|   TEXAS INSTRUMENTS INCORPORATED
|   Standard Linear and Logic
|   IBIS Model of SN74LVTH162373
|   3.3-V ABT 16-BIT TRANSPARENT D-TYPE LATCHES
|   WITH 3-STATE OUTPUTS
|   TSSOP 48-pin package (DGG)
|   SSOP 48-pin package (DL)
[IBIS Ver]   3.2
[Comment char]   |_char
[File Name]   sn74lvth162373.ibs
[File Rev]   1.1 | a_die
[Date]   10/08/03
[Source]   File originated at Texas Instruments, Inc
[Notes]   The following is an IBIS list for SN74LVTH162373.
|   - All test data contained in this file are derived from
|   actual measurement.
|   - Non-monotonic data in ground-clamp due to bus-hold
|   - Power clamp data deleted in input models.
|   - Non-monotonic data in pullup data due to resistor at output.
|   - End point warning due to AC and DC mismatch.
|   - File created by Nobuhisa Ohtsubo, TIJ SLL Product Engineering.
|*   Property of Texas Instruments Incorporated.  Unauthorized   *
|*   reproduction and/or distribution is strictly prohibited.   *
|*   This product is protected under copyright law.   *
|*   Created 1998, (C) Copyright 1998, Texas Instruments Inc.,   *
|*   All Rights Reserved   *
|*   UNLESS THERE IS A SIGNED, WRITTEN AGREEMENT TO THE   *
|*   CONTRARY, TEXAS INSTRUMENTS ("TI") IS PROVIDING THE SPICE   *
|*   MODELS "AS IS" AND WITHOUT ANY WARRANTY, EXPRESSED OR   *
|*   IMPLIED.  TI assumes no liability for:   *
|*   1) the accuracy of the IBIS models provided to your   *
|*   company;   *
|*   2) the proper functioning of these IBIS models in your   *
|*   design or for any resulting applications; or   *
|*   3) infringement of patents, copyrights or intellectual   *
|*   property rights resulting from your use of these   *
|*   IBIS models.   *
|*   TI provides IBIS Models as a service to our customers.   *
|*   You and your company shall not distribute, sell or give   *
|*   these models to anyone else without prior written   *
|*   permission from TI.   *
|*   TI reserves the right to make changes to our products or   *
|*   to discontinue any semiconductor product or service   *
|*   without notice, and advises our customers to obtain the   *
|*   latest version of relevant information to verify, before   *
|*   placing orders, that the information being relied on is   *
|*   current.   *
|*   Please be aware that your receipt and use of the IBIS   *
|*   information provided shall serve as acceptance of these   *
|*   terms and conditions.  If you do not accept these terms,   *
|*   you should return or destroy the IBIS models and any   *
|*   other accompanying information immediately.   *
|   TSSOP PACKAGE (DGG)
[Component]   LVTH162373_DGG
[manufacturer]   Texas Instruments, Inc.
[Package]
|   typ   min   max
R_pkg   0.044   0.038   0.051
L_pkg   3.019nH   2.486nH   4.099nH
C_pkg   0.507pF   0.334pF   0.809pF
[Pin] signal_name   model_name   R_pin   L_pin   C_pin
1   1NOE   LVTH162373_CTRL  0.041   4.017nH   0.759pF
2   1Q1   LVTH162373_OUT   0.042   3.737nH   0.792pF
3   1Q2   LVTH162373_OUT   0.042   3.48nH   0.661pF
4   GND   GND   0.038   3.131nH   0.575pF
5   1Q3   LVTH162373_OUT   0.047   3.122nH   0.566pF
6   1Q4   LVTH162373_OUT   0.043   2.948nH   0.504pF
7   VCC   POWER   0.045   2.845nH   0.397pF
8   1Q5   LVTH162373_OUT   0.049   2.835nH   0.394pF
9   1Q6   LVTH162373_OUT   0.048   2.715nH   0.378pF
10   GND   GND   0.050   2.664nH   0.363pF
11   1Q7   LVTH162373_OUT   0.050   2.585nH   0.348pF
12   1Q8   LVTH162373_OUT   0.049   2.55nH   0.337pF
13   2Q1   LVTH162373_OUT   0.049   2.541nH   0.336pF
14   2Q2   LVTH162373_OUT   0.050   2.574nH   0.348pF
15   GND   GND   0.049   2.618nH   0.359pF
16   2Q3   LVTH162373_OUT   0.046   2.671nH   0.375pF
17   2Q4   LVTH162373_OUT   0.045   2.754nH   0.389pF
18   VCC   POWER   0.044   2.823nH   0.450pF
19   2Q5   LVTH162373_OUT   0.042   2.968nH   0.503pF
20   2Q6   LVTH162373_OUT   0.051   3.108nH   0.535pF
21   GND   GND   0.042   3.175nH   0.587pF
22   2Q7   LVTH162373_OUT   0.041   3.449nH   0.678pF
23   2Q8   LVTH162373_OUT   0.044   3.766nH   0.804pF
24   2NOE   LVTH162373_CTRL  0.043   4.065nH   0.761pF
25   2LE   LVTH162373_CTRL  0.041   3.994nH   0.757pF
26   2D8   LVTH162373_IN   0.039   3.649nH   0.789pF
27   2D7   LVTH162373_IN   0.038   3.362nH   0.660pF
28   GND   GND   0.038   3.082nH   0.574pF
29   2D6   LVTH162373_IN   0.044   2.99nH   0.522pF
30   2D5   LVTH162373_IN   0.041   2.917nH   0.495pF
31   VCC   POWER   0.043   2.82nH   0.448pF
32   2D4   LVTH162373_IN   0.043   2.699nH   0.385pF
33   2D3   LVTH162373_IN   0.045   2.628nH   0.372pF
34   GND   GND   0.046   2.556nH   0.356pF
35   2D2   LVTH162373_IN   0.046   2.495nH   0.344pF
36   2D1   LVTH162373_IN   0.047   2.487nH   0.334pF
37   1D8   LVTH162373_IN   0.047   2.49nH   0.335pF
38   1D7   LVTH162373_IN   0.046   2.486nH   0.343pF
39   GND   GND   0.045   2.566nH   0.356pF
40   1D6   LVTH162373_IN   0.044   2.639nH   0.374pF
41   1D5   LVTH162373_IN   0.043   2.701nH   0.386pF
42   VCC   POWER   0.043   2.817nH   0.450pF
43   1D4   LVTH162373_IN   0.041   2.935nH   0.501pF
44   1D3   LVTH162373_IN   0.047   3.035nH   0.529pF
45   GND   GND   0.043   3.171nH   0.589pF
46   1D2   LVTH162373_IN   0.040   3.415nH   0.682pF
47   1D1   LVTH162373_IN   0.043   3.741nH   0.809pF
48   1LE   LVTH162373_CTRL  0.044   4.099nH   0.764pF
|   SSOP PACKAGE (DL)
[Component]   LVTH162373_DL
[manufacturer]   Texas Instruments,Inc.
[Package]
|   typ   min   max
R_pkg   0.048   0.038   0.053
L_pkg   6.046nH   5.084nH   7.968nH
C_pkg   0.813pF   0.569pF   1.157pF
[Pin] signal_name   model_name   R_pin   L_pin   C_pin
1   1NOE   LVTH162373_CTRL  0.046   7.968nH   1.017pF
2   1Q1   LVTH162373_OUT   0.044   7.299nH   1.157pF
3   1Q2   LVTH162373_OUT   0.043   6.765nH   1.058pF
4   GND   GND   0.041   6.269nH   0.933pF
5   1Q3   LVTH162373_OUT   0.038   5.856nH   0.829pF
6   1Q4   LVTH162373_OUT   0.046   5.802nH   0.790pF
7   VCC   POWER   0.050   5.656nH   0.738pF
8   1Q5   LVTH162373_OUT   0.053   5.5nH   0.643pF
9   1Q6   LVTH162373_OUT   0.052   5.304nH   0.606pF
10   GND   GND   0.053   5.189nH   0.583pF
11   1Q7   LVTH162373_OUT   0.051   5.084nH   0.569pF
12   1Q8   LVTH162373_OUT   0.053   5.862nH   0.833pF
13   2Q1   LVTH162373_OUT   0.053   5.862nH   0.833pF
14   2Q2   LVTH162373_OUT   0.051   5.084nH   0.569pF
15   GND   GND   0.053   5.189nH   0.583pF
16   2Q3   LVTH162373_OUT   0.052   5.304nH   0.606pF
17   2Q4   LVTH162373_OUT   0.053   5.5nH   0.643pF
18   VCC   POWER   0.050   5.656nH   0.738pF
19   2Q5   LVTH162373_OUT   0.046   5.802nH   0.790pF
20   2Q6   LVTH162373_OUT   0.038   5.856nH   0.829pF
21   GND   GND   0.041   6.269nH   0.933pF
22   2Q7   LVTH162373_OUT   0.043   6.765nH   1.058pF
23   2Q8   LVTH162373_OUT   0.044   7.299nH   1.157pF
24   2NOE   LVTH162373_CTRL  0.046   7.968nH   1.017pF
25   2LE   LVTH162373_CTRL  0.046   7.968nH   1.017pF
26   2D8   LVTH162373_IN   0.044   7.299nH   1.157pF
27   2D7   LVTH162373_IN   0.043   6.765nH   1.058pF
28   GND   GND   0.041   6.269nH   0.933pF
29   2D6   LVTH162373_IN   0.038   5.856nH   0.829pF
30   2D5   LVTH162373_IN   0.046   5.802nH   0.790pF
31   VCC   POWER   0.050   5.656nH   0.738pF
32   2D4   LVTH162373_IN   0.053   5.5nH   0.643pF
33   2D3   LVTH162373_IN   0.052   5.304nH   0.606pF
34   GND   GND   0.053   5.189nH   0.583pF
35   2D2   LVTH162373_IN   0.051   5.084nH   0.569pF
36   2D1   LVTH162373_IN   0.053   5.862nH   0.833pF
37   1D8   LVTH162373_IN   0.053   5.862nH   0.833pF
38   1D7   LVTH162373_IN   0.051   5.084nH   0.569pF
39   GND   GND   0.053   5.189nH   0.583pF
40   1D6   LVTH162373_IN   0.052   5.304nH   0.606pF
41   1D5   LVTH162373_IN   0.053   5.5nH   0.643pF
42   VCC   POWER   0.005   5.656nH   0.738pF
43   1D4   LVTH162373_IN   0.046   5.802nH   0.790pF
44   1D3   LVTH162373_IN   0.038   5.856nH   0.829pF
45   GND   GND   0.041   6.269nH   0.933pF
46   1D2   LVTH162373_IN   0.043   6.765nH   1.058pF
47   1D1   LVTH162373_IN   0.044   7.299nH   1.157pF
48   1LE   LVTH162373_CTRL  0.046   7.967nH   1.017pF
[Model Selector]   LVTH162373_IN
LVTH162373_IN_28   2.8-V Vcc Input Model
LVTH162373_IN_33   3.3-V Vcc Input Model
[Model Selector]   LVTH162373_CTRL
LVTH162373_CTRL_28   2.8-V Vcc Input Model
LVTH162373_CTRL_33   3.3-V Vcc Input Model
[Model Selector]   LVTH162373_OUT
LVTH162373_OUT_28   2.8-V Vcc Output Model
LVTH162373_OUT_33   3.3-V Vcc Output Model
| Models and submodels in the file (6): LVTH162373_OUT_28 (3-state), LVTH162373_CTRL_28 (Input), LVTH162373_IN_28 (Input), LVTH162373_OUT_33 (3-state), LVTH162373_CTRL_33 (Input), LVTH162373_IN_33 (Input)
